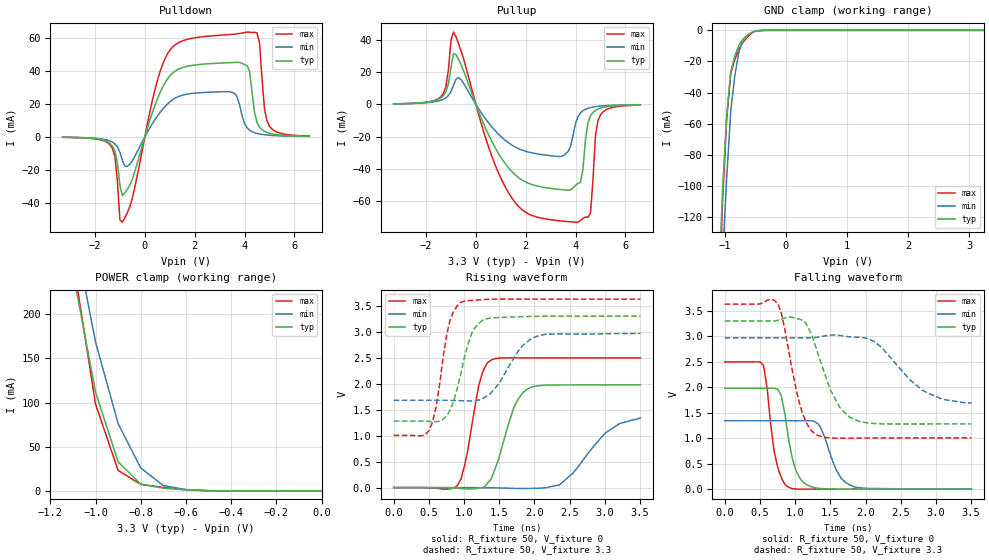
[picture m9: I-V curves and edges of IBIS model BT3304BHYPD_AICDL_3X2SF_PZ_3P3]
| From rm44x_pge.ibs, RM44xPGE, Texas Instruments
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|   Model Cell BT3304BHYPD_AICDL_3X2SF_PZ_3P3
|BT3304BHYPD_AICDL_3X2SF_PZ_3P3
[Model]   BT3304BHYPD_AICDL_3X2SF_PZ_3P3
Model_type   I/O
Polarity   Non-Inverting
Enable   Active-Low
Vinl =  1.15
Vinh =  1.55
Cref =  15.0001pF
Rref =  101.0000M
Vref =  0V
Vmeas =  1.65
C_comp   1.2p   1.2p   1.2p
[Model Spec]
Vinl   1.15   1.02   1.28
Vinh   1.55   1.45   1.65
[Temperature Range]   25   155   -40
[Voltage Range]   3.3   2.97   3.63
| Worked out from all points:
|   slope of the pulldown table from 0 to 0.495 V, typ, clamps not added: 22 ohm
|   slope of the pullup table from 0 to 0.495 V, typ, clamps not added: 26.9 ohm
|   GND clamp passes 1 mA (typ) near -0.53 V on its own axis
|   POWER clamp passes 1 mA (typ) near -0.59 V on its own axis
|   rising waveform, R_fixture 50, V_fixture 0: 20-80 % time 273ps typ, 493ps min, 197ps max; typ from 0 V to 1.98 V
|   rising waveform, R_fixture 50, V_fixture 3.3: 20-80 % time 234ps typ, 363ps min, 182ps max; typ from 1.28 V to 3.3 V
|   falling waveform, R_fixture 50, V_fixture 0: 20-80 % time 165ps typ, 226ps min, 141ps max; typ from 1.98 V to 0 V
|   falling waveform, R_fixture 50, V_fixture 3.3: 20-80 % time 334ps typ, 534ps min, 237ps max; typ from 3.3 V to 1.28 V
[POWER_clamp]
|   voltage   I(typ)   I(min)   I(max)
-3.3V     4.054A     4.63A      4.887A
-1.1V     248.3mA    301mA      262.7mA
-1.067V   202.9mA    256.9mA    207.9mA
-1.033V   157.5mA    212.7mA    153.1mA
-1V       112.1mA    168.6mA    98.29mA
-900mV    32.88mA    76.23mA    23.22mA
-800mV    7.706mA    25.95mA    7.477mA
-700mV    3.034mA    6.039mA    3.991mA
-600mV    1.088mA    1.528mA    1.425mA
-500mV    187.1uA    369uA      203.4uA
0V        443pA      6.159nA    417pA
[Pulldown]
|   voltage   I(typ)   I(min)   I(max)
-3.3V     -289uA     -253.9uA   -287.1uA
-1.4V     -4mA       -2.489mA   -4.76mA
-1.2V     -8.69mA    -4.261mA   -12.05mA
-1V       -29.49mA   -9.376mA   -50.19mA
-900mV    -35.6mA    -14.42mA   -51.59mA
1V        36.78mA    21.07mA    52.28mA
3.5V      44.86mA    26.91mA    61.93mA
4.1V      42.98mA    5.455mA    63.29mA
4.6V      5.887mA    1.718mA    56.92mA
4.8V      3.323mA    1.257mA    16.92mA
5V        2.171mA    957.9uA    6.458mA
6.6V      331.3uA    239.5uA    466.8uA
[Pullup]
|   voltage   I(typ)   I(min)   I(max)
-3.3V     325.3uA    297.6uA    301.6uA
-1.4V     4.042mA    2.556mA    4.795mA
-1.2V     7.932mA    4.062mA    11.12mA
-900mV    31.45mA    11.76mA    44.76mA
1.4V      -40.91mA   -24.77mA   -56.99mA
3.4V      -52.76mA   -32.29mA   -72.18mA
4V        -50.08mA   -11.8mA    -72.98mA
4.2V      -48.37mA   -5.201mA   -71.98mA
4.6V      -7.019mA   -1.989mA   -67.23mA
4.8V      -3.708mA   -1.414mA   -19.03mA
5V        -2.349mA   -1.055mA   -6.475mA
6.6V      -340.9uA   -258.1uA   -448.7uA
[GND_clamp]
|   voltage   I(typ)   I(min)   I(max)
-3.3V     -3.25A     -2.875A    -4.945A
-1.1V     -166.9mA   -205mA     -187mA
-1.033V   -102.7mA   -146.7mA   -110.1mA
-966.7mV  -55.96mA   -95.69mA   -57.02mA
-900mV    -26.55mA   -52.03mA   -27.8mA
-833.3mV  -16.49mA   -29.28mA   -18.77mA
-766.7mV  -9.539mA   -13.91mA   -12.07mA
-700mV    -5.69mA    -5.924mA   -7.706mA
-566.7mV  -1.567mA   -1.63mA    -2.054mA
-500mV    -402.3uA   -594.3uA   -459.7uA
-366.7mV  -18.7uA    -59.25uA   -17.4uA
3.233V    423.5pA    4.09uA     323pA
[Ramp]
| variable   typ   min   max
dV/dt_f   1.260452/0.3438406n  0.8110476/0.5624008n   1.639064/0.2455425n
dV/dt_r   1.203253/0.2763702n  0.8165587/0.5016654n   1.517691/0.1983433n
R_load = 50
[Rising Waveform]
R_fixture = 50
V_fixture = 0
V_fixture_min = 0
V_fixture_max = 0
|   time   V(typ)   V(min)   V(max)
0s        -5.703uV   -2.799uV   -3.362uV
904ps     -13.01mV   203.3uV    38.38mV
1.008ns   -23.7mV    251.7uV    427.7mV
1.256ns   427.7uV    -1.944mV   2.193V
1.408ns   247.7mV    -4.996mV   2.471V
1.708ns   1.546V     -14.43mV   2.499V
1.904ns   1.904V     -16.2mV    2.498V
2.356ns   1.977V     54.01mV    2.497V
3.008ns   1.978V     1.054V     2.497V
3.504ns   1.979V     1.342V     2.497V
[Rising Waveform]
R_fixture = 50
V_fixture = 3.3
V_fixture_min = 2.97
V_fixture_max = 3.63
|   time   V(typ)   V(min)   V(max)
0s        1.281V     1.682V     1.005V
504ps     1.275V     1.682V     1.103V
604ps     1.27V      1.682V     1.56V
756ps     1.391V     1.681V     2.965V
804ps     1.491V     1.68V      3.241V
956ps     2.205V     1.673V     3.57V
1.108ns   2.969V     1.668V     3.605V
1.284ns   3.241V     1.733V     3.621V
1.968ns   3.297V     2.884V     3.63V
3.504ns   3.3V       2.969V     3.63V
[Falling Waveform]
R_fixture = 50
V_fixture = 0
V_fixture_min = 0
V_fixture_max = 0
|   time   V(typ)   V(min)   V(max)
0s        1.979V     1.342V     2.498V
552ps     1.979V     1.342V     2.425V
704ps     1.981V     1.342V     732.4mV
804ps     1.835V     1.342V     225.1mV
904ps     1.011V     1.342V     39.22mV
1.056ns   240.9mV    1.342V     304.3uV
1.256ns   35.03mV    1.338V     654.2uV
1.656ns   2.463mV    210.1mV    465.3uV
1.836ns   1.295mV    46.59mV    446.6uV
3.504ns   292.6uV    543.2uV    26.45uV
[Falling Waveform]
R_fixture = 50
V_fixture = 3.3
V_fixture_min = 2.97
V_fixture_max = 3.63
|   time   V(typ)   V(min)   V(max)
0s        3.3V       2.97V      3.63V
756ps     3.311V     2.97V      3.636V
804ps     3.333V     2.97V      3.456V
1.108ns   3.312V     2.97V      1.474V
1.308ns   2.727V     2.979V     1.061V
1.508ns   1.932V     3.023V     1.006V
1.772ns   1.413V     2.99V      1.002V
2.164ns   1.286V     2.853V     1.005V
2.876ns   1.28V      1.89V      1.006V
3.504ns   1.281V     1.693V     1.006V
